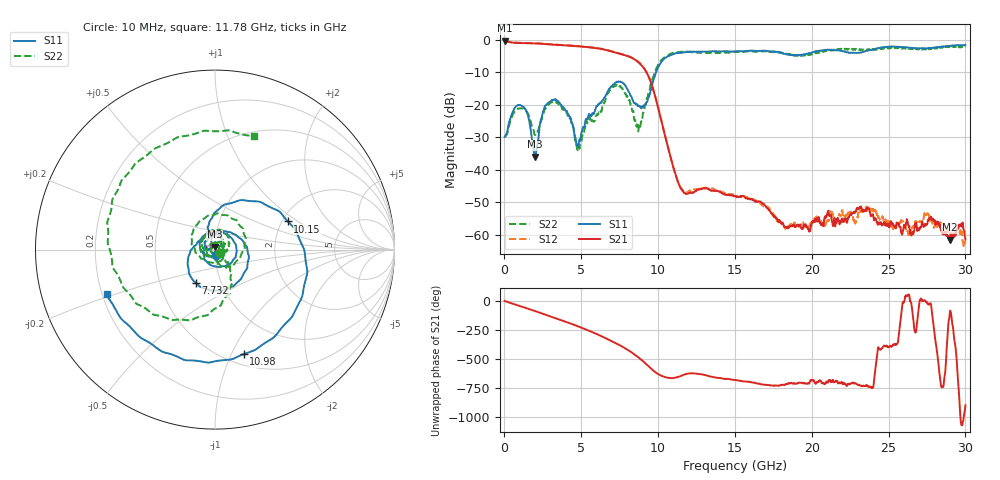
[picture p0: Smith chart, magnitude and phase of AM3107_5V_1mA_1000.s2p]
# Hz S DB R 50.0
!freq dBS11 angS11 dBS21 angS21 dBS12 angS12 dBS22 angS22
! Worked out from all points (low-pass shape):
!   1601 points, 10 MHz to 30 GHz, reference 50 ohm
!   highest |S21| = -0.21 dB at 10 MHz (marker M1); lowest = -61.5 dB at 28.99 GHz (marker M2)
!   |S21| within 3 dB of the highest: start of sweep to 6.722 GHz
!   lowest |S11| = -35.9 dB at 1.978 GHz (marker M3), VSWR 1.03, Z = 49.9 + j1.59 ohm
!   |S11| at or under -10 dB: start of sweep to 9.859 GHz
!   |S22| runs from -34.2 to -1.8 dB; largest |S21 - S12| = 0.012
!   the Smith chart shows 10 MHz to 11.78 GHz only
!   S11 on the Smith chart (normalised r, x): 10 MHz: 1.01, -0.06; 7.732 GHz: 0.76, -0.30; 10.15 GHz: 2.15, +0.83; 10.98 GHz: 0.61, -1.11; 11.78 GHz: 0.22, -0.19
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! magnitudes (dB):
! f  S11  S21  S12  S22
! 10 MHz  -29.9  -0.2  -0.1  -29.7
! 1.116 GHz  -20.2  -0.9  -0.9  -21.0
! 1.978 GHz  -35.9  -1.0  -0.9  -29.3
! 2.559 GHz  -21.6  -1.2  -1.1  -22.3
! 3.178 GHz  -18.5  -1.4  -1.4  -19.1
! 4.715 GHz  -32.4  -1.9  -1.8  -33.3
! 5.015 GHz  -28.5  -2.0  -1.9  -31.0
! 6.945 GHz  -14.3  -3.5  -3.4  -14.9
! 7.732 GHz  -13.4  -4.5  -4.4  -15.6
! 8.726 GHz  -20.1  -6.9  -6.7  -27.7
! 10.02 GHz  -8.3  -21.2  -21.1  -7.5
! 10.15 GHz  -7.2  -23.7  -23.6  -6.6
! 10.98 GHz  -4.4  -39.0  -39.0  -3.9
! 11.78 GHz  -3.7  -47.4  -47.0  -3.5
! 15.01 GHz  -3.5  -48.0  -47.9  -3.6
! 20.01 GHz  -3.8  -56.1  -56.8  -4.4
! 23.08 GHz  -3.9  -51.7  -53.0  -3.0
! 25.01 GHz  -2.0  -57.5  -57.0  -2.6
! 26.31 GHz  -2.3  -57.3  -59.7  -2.7
! 27.49 GHz  -2.6  -56.7  -53.8  -2.6
! 28.99 GHz  -1.9  -61.5  -59.7  -2.2
! 30 GHz  -1.5  -61.5  -62.6  -1.9
